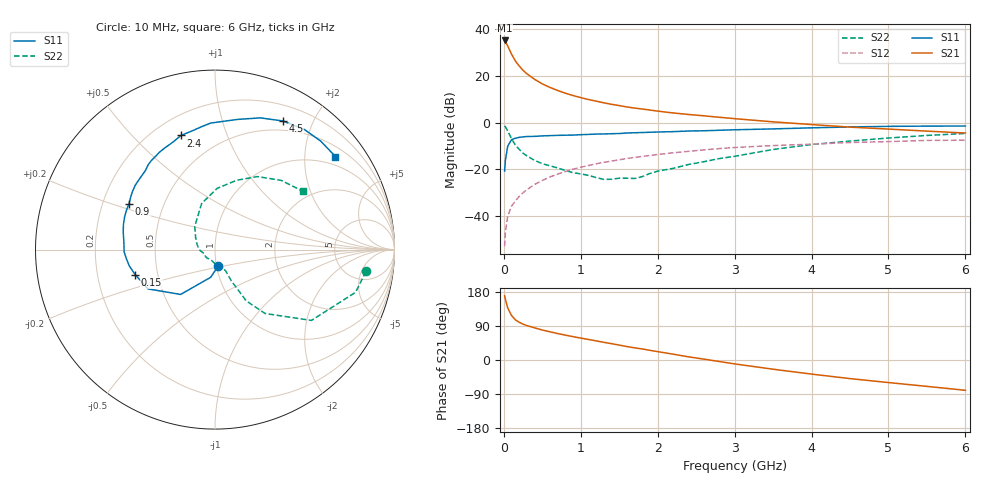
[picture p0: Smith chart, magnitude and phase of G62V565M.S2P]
! SIEMENS Small Signal Semiconductors
! BFG193
! Si NPN RF Bipolar Junction Transistor in SOT223
! VCE = 2.5 V  IC = 65 mA
! Common Emitter S-Parameters:  August  1996
# GHz  S  MA  R  50
!  f  S11  S21  S12  S22
! GHz  MAG  ANG  MAG  ANG  MAG  ANG  MAG  ANG
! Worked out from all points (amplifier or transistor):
!   36 points, 10 MHz to 6 GHz, reference 50 ohm
!   highest |S21| = 35.1 dB at 10 MHz (marker M1)
!   |S21| within 3 dB of that: start of sweep to 59.35 MHz
!   unconditionally stable (mu >= 1): start of sweep to 10.64 MHz; 297 MHz to 2.524 GHz
!   at 250 MHz: K = 0.98, MSG = 26.1 dB, |S12| = -29.9 dB
!   at 1.4 GHz: K = 1.07, MAG = 10.5 dB, |S12| = -16.4 dB
!   at 6 GHz: K = 0.93, MSG = 1.5 dB, |S12| = -7.5 dB
!   S11 on the Smith chart (normalised r, x): 10 MHz: 1.02, -0.19; 150 MHz: 0.37, -0.13; 900 MHz: 0.31, +0.23; 2.4 GHz: 0.31, +0.70; 4.5 GHz: 0.38, +1.59; 6 GHz: 0.74, +2.75
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0.01  0.0923 -78.4  57.09 169.5  0.0023 79.7  0.8498 -8.2
0.02  0.1566 -99.0  54.39 160.3  0.0045 76.1  0.8186 -16.9
0.05  0.3149 -127.5  43.59 137.5  0.0101 67.7  0.6665 -36.3
0.1  0.4327 -149.6  29.08 117.5  0.0164 66.7  0.4524 -51.9
0.15  0.4658 -162.5  20.82 106.0  0.0214 66.2  0.3338 -58.7
0.2  0.486 -169.2  16.21 99.6  0.0266 68.6  0.269 -59.9
0.25  0.4972 -174.5  13.12 94.6  0.0319 69.1  0.2217 -61.4
0.3  0.5063 -178.6  11.09 90.8  0.0371 70.1  0.1957 -62.4
0.4  0.5101 174.8  8.417 84.8  0.048 70.1  0.1562 -62.9
0.5  0.5213 168.8  6.749 79.1  0.0582 68.7  0.1331 -63.3
0.6  0.5291 164.6  5.663 74.4  0.0693 67.9  0.1197 -65.7
0.7  0.5358 159.9  4.87 69.8  0.0797 66.3  0.1078 -69.8
0.9  0.5432 151.8  3.8 61.6  0.1017 62.6  0.0854 -76.8
1.1  0.5617 145.0  3.125 54.2  0.1217 58.7  0.0749 -93.3
1.3  0.5745 138.1  2.655 46.6  0.1422 54.6  0.0615 -112.0
1.6  0.6019 128.2  2.165 35.5  0.1715 47.5  0.0651 -146.1
2.2  0.6433 111.3  1.614 15.4  0.2272 33.6  0.1056 162.7
2.4  0.6637 106.6  1.497 8.4  0.2441 29.3  0.1277 147.9
3.5  0.736 80.2  1.042 -24.3  0.324 1.6  0.2677 106.1
4.5  0.8102 62.2  0.803 -49.1  0.3768 -18.7  0.4046 72.7
5.5  0.844 45.7  0.66 -69.6  0.4186 -42.1  0.5336 46.3
6  0.848 37.7  0.601 -80.0  0.4217 -55.5  0.5878 33.5
